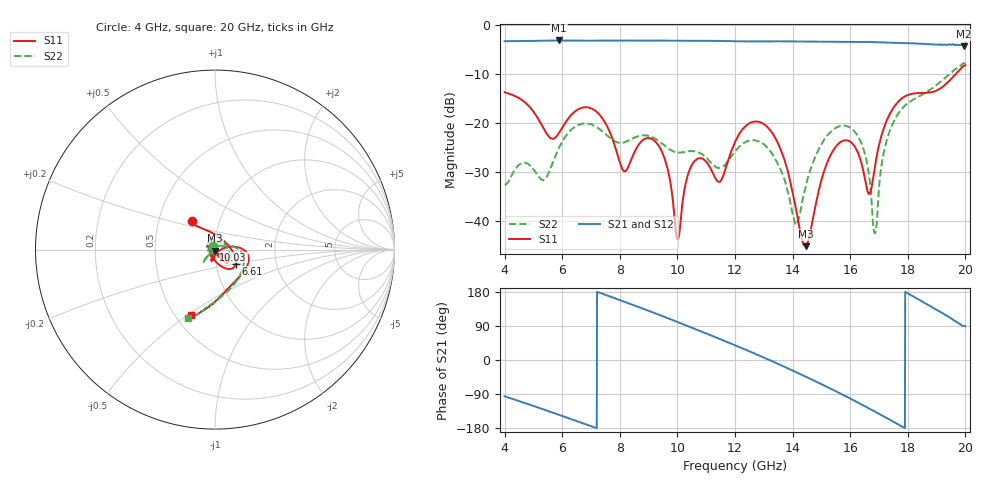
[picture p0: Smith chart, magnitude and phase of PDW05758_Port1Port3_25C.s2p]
! "!Agilent Technologies,E8361A,US43140610,A.07.50.67"
!Agilent E8361A: A.07.50.67
! "!Date: Friday, February 28, 2014 12:27:08"
! "!Correction: S11(Full 2 Port(1,2)) "
! "!S21(Full 2 Port(1,2)) "
! "!S12(Full 2 Port(1,2)) "
! "!S22(Full 2 Port(1,2)) "
! "!S2P File: Measurements: S11, S21, S12, S22:"
!Power divider measured mounted on 10mil RO4350 with coaxial edge launch connectors.  Coaxial connectors have been gated out.  Unused port was externally terminated
!with coaxial termination.  Measurement reference plane placed at the part edge.  The loss of the test board and connectors has been removed.
!Port one = common port
!Port two = output port
# GHz S MA R 50
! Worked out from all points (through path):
!   1601 points, 4 GHz to 20 GHz, reference 50 ohm
!   highest |S21| = -3.16 dB at 5.89 GHz (marker M1); lowest = -4.4 dB at 19.95 GHz (marker M2)
!   lowest |S11| = -45.2 dB at 14.46 GHz (marker M3), VSWR 1.01, Z = 50.1 - j0.545 ohm
!   |S11| at or under -10 dB: start of sweep to 19.67 GHz
!   |S22| runs from -42.6 to -7.8 dB; largest |S21 - S12| = 0.03
!   S11 on the Smith chart (normalised r, x): 4 GHz: 0.73, +0.24; 6.61 GHz: 1.24, -0.20; 10.03 GHz: 0.99, -0.00; 20 GHz: 0.60, -0.52
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4  0.2059 129.5  0.683 -95.8  0.6829 -95.8  0.0234 122.4
5.89  0.07899 15.3  0.6952 -144.7  0.695 -144.8  0.05578 -45.8
6.61  0.1403 -34.6  0.6926 -164.1  0.6908 -164.0  0.09649 -29.3
6.67  0.142 -37.0  0.6921 -165.6  0.6901 -165.6  0.09731 -28.5
8.15  0.03206 -154.7  0.6938 153.8  0.6909 153.9  0.06318 45.6
9.34  0.05889 100.1  0.693 120.0  0.6926 119.9  0.06563 95.8
10.03  0.006567 -179.2  0.6906 99.6  0.6908 99.7  0.04964 134.5
10.53  0.03827 -122.6  0.6893 84.7  0.6886 84.6  0.05141 152.6
11.47  0.02502 -78.9  0.6868 55.6  0.6863 55.6  0.03439 101.1
12  0.06363 -32.0  0.6817 38.8  0.6817 38.7  0.05114 49.6
13.29  0.07887 -53.5  0.68 -3.3  0.68 -3.2  0.04844 32.1
14.11  0.01358 -71.0  0.678 -31.8  0.6768 -31.8  0.009058 118.9
14.46  0.005488 -82.9  0.6777 -44.2  0.6779 -44.2  0.02271 -160.9
14.67  0.009265 -86.1  0.6761 -51.8  0.6756 -51.9  0.03684 -147.3
15.33  0.04741 -97.2  0.6734 -76.1  0.6707 -76.2  0.08101 -134.4
16.1  0.06031 -110.8  0.6725 -105.6  0.6715 -105.6  0.08486 -135.2
16.64  0.01888 -60.4  0.6682 -127.2  0.6689 -127.2  0.03114 -138.6
16.86  0.0358 2.6  0.6672 -136.3  0.6674 -136.2  0.007429 -56.0
17.34  0.1172 7.5  0.6608 -156.1  0.6617 -155.9  0.07736 14.6
18.52  0.2022 -36.1  0.6407 153.5  0.639 153.5  0.1957 -42.2
19.95  0.3828 -108.2  0.6041 89.8  0.5938 87.5  0.4053 -110.3
20  0.3888 -109.8  0.6054 89.3  0.5883 87.0  0.409 -111.3
